FUNCTION_BLOCK FB_Visu
VAR_INPUT
	(***** Sensors to detect boxes *****)
	bBarrierSensor				AT %I*: BOOL;	// True if barrier sensor detects a box
	bMetalSensor				AT %I*: BOOL;	// True if metal sensor detects a metal box
	bPlasticSensor				AT %I*: BOOL;	// True if plastic sensor detects a box
	
	bError						: BOOL;			// True if modules have errors
(***** Axis variables *****)
	lrAxisVelo					: LREAL;
	
(***** State of machine elements *****)
	bComprAirEnabled			: BOOL;			// True if compressed air is enabled
	bPowerEnabled				: BOOL;			// True if power supply is enabled
	bMainAxisMoves				: BOOL;			// True if main axis is moving
	bMetalAxisMoves				: BOOL;			// True if metal axis is moving
	bPlasticAxisMoves			: BOOL;			// True if plastic axis is moving
	bClampToWork				: BOOL;			// True if clamp cylinder moves to work position
	bBarrierToWork				: BOOL;			// True if barrier cylinder moves to work position
	bMetalToWork				: BOOL;			// True if metal cylinder moves to work position
	bPlasticToWork				: BOOL;			// True if plastic cylinder moves to work position
(***** Error *****)
	bClampError					: BOOL;			// True if clamp cylinder has an error
	sClampErrMsg				: STRING;		// Error message of clamp cylinder
	bMetalCylError				: BOOL;			// True if metal cylinder has an error
	sMetalErrMsg				: STRING;		// Error message of metal cylinder
	bPlasticCylError			: BOOL;			// True if plastic cylinder has an error
	sPlasticErrMsg				: STRING;		// Error message of plastic cylinder
	nMainAxisErrorId			: DWORD;		// Error id of main axis
	nMetalAxisErrorId			: DWORD;		// Error id of metal axis
	nPlasticAxisErrorId			: DWORD;		// Error id of plastic axis
	
(***** PS_PackML_StateMachine *****)
	bStarted					: BOOL;			// True if state machine is in state EXECUTE
	bStopped					: BOOL;			// True if state machine is in state STOPPED
	bReset						: BOOL;			// True if state machine is in state RESETTING
	bAborted					: BOOL;			// True if state machine is in state ABORTED
	bIdle						: BOOL;			// True if state machine is in state IDLE
	bAuto						: BOOL;			// True if state machine is in mode AUTOMATIC
	bSemi						: BOOL;			// True if state machine is in mode SEMIAUTOMATIC
	bManual						: BOOL;			// True if state machine is in mode MANUAL
	bMaintenance				: BOOL;			// True if state machine is in mode MAINTENANCE
	bStartButtonOff				: BOOL;			// To turn off start button

(***** Buttons of visualisation - inputs *****)
		(* State buttons *)
	bButtonPowerIn				: BOOL;			// Input signal of power button
	bButtonComprAirIn			: BOOL;			// Input signal of compressed air button
	bButtonStartIn				: BOOL;			// Input signal of start button
	bButtonStopIn				: BOOL;			// Input signal of stop button
	bButtonResetIn				: BOOL;			// Input signal of reset button
	bButtonAbortIn				: BOOL;			// Input signal of abort button
		(* Mode buttons *)
	bButtonAutoIn				: BOOL;			// Input signal of automatic button
	bButtonSemiIn				: BOOL;			// Input signal of semi-automatic button
	bButtonManuIn				: BOOL;			// Input signal of manual button
	bButtonMaintenanceIn		: BOOL;			// Input signal of maintenance button
		(* Axis buttons *)
	bButtonMainFwIn				: BOOL;			// Input signal of button to move main axis forwards
	bButtonMainBwIn				: BOOL;			// Input signal of button to move main axis backwards
	bButtonMetalFwIn			: BOOL;			// Input signal of button to move metal axis forwards
	bButtonMetalBwIn			: BOOL;			// Input signal of button to move metal axis backwards
	bButtonPlasticFwIn			: BOOL;			// Input signal of button to move plastic axis forwards
	bButtonPlasticBwIn			: BOOL;			// Input signal of button to move plastic axis backwards
		(* Cylinder buttons *)
	bButtonClampToWorkIn		: BOOL;			// Input signal of button to move clamp cylinder
	bButtonBarrierToWorkIn		: BOOL;			// Input signal of button to move barrier cylinder
	bButtonMetalToWorkIn		: BOOL;			// Input signal of button to move metal cylinder
	bButtonPlasticToWorkIn		: BOOL;			// Input signal of button to move plastic cylinder
END_VAR
VAR_OUTPUT
	lrYClamp					AT %Q*: LREAL;					// Y-Coordinate of clamp cylinder
	lrYBarrier					AT %Q*: LREAL;					// Y-Coordinate of barrier cylinder
	lrYMetal					AT %Q*: LREAL;					// Y-Coordinate of metal cylinder
	lrYPlastic					AT %Q*: LREAL;					// Y-Coordinate of plastic cylinder
	aBoxX						AT %Q*: ARRAY[1..4] OF LREAL;	// X-Coordinates of boxes
	aBoxY						AT %Q*: ARRAY[1..4] OF LREAL;	// Y-Coordinates of boxes
	
(***** Buttons of visualisation - outputs *****)
		(* State buttons *)
	bButtonPowerOut				: BOOL;			// To turn on and off the machine
	bButtonComprAirOut			: BOOL;			// To enable compressed air
	bButtonStartOut				: BOOL;			// To change state into state START
	bButtonStopOut				: BOOL;			// To change state into state STOP
	bButtonResetOut				: BOOL;			// To change state into state RESET
	
		(* Mode buttons *)
	bButtonAutoOut				: BOOL;			// To change mode into mode AUTOMATIC		
	bButtonSemiOut				: BOOL;			// To change mode into mode SEMI-AUTOMATIC	
	bButtonManuOut				: BOOL;			// To change mode into mode MANAUL	
	bButtonMaintenanceOut		: BOOL;			// To change mode into mode MAINTENANCE	
	
		(* Axis buttons *)
	bButtonMainFwOut			: BOOL;			// To move main axis forwards
	bButtonMainBwOut			: BOOL;			// To move main axis backwards
	bButtonMetalFwOut			: BOOL;			// To move metal axis forwards
	bButtonMetalBwOut			: BOOL;			// To move metal axis backwards
	bButtonPlasticFwOut			: BOOL;			// To move plastic axis forwards
	bButtonPlasticBwOut			: BOOL;			// To move plastic axis backwards
	
		(* Cylinder buttons *)
	bButtonClampToWorkOut		: BOOL;			// To move manually clamp cylinder to work position
	bButtonBarrierToWorkOut		: BOOL;			// To move manually barrier cylinder to work position
	bButtonMetalToWorkOut		: BOOL;			// To move manually metal cylinder to work position
	bButtonPlasticToWorkOut		: BOOL;			// To move manually plastic cylinder to work position
END_VAR
VAR
	nBoxesLast					: INT;						// Box on last position of main belt
	aBoxMetalMove				: ARRAY[1..4] OF BOOL;		// bBoxMetalMove[1] is true, if box 1 is moved by metal cylinder
	aBoxMetalFree				: ARRAY[1..4] OF BOOL;		// bBoxMetalFree[1] is true, if any box blockades the metal belt
	aBoxPlasticMove				: ARRAY[1..4] OF BOOL;		// bBoxPlasticMove[1] is true, if box 1 is moved by plastic cylinder
	aBoxPlasticFree				: ARRAY[1..4] OF BOOL;		// bBoxMetalFree[1] is true, if any box blockades the plastic belt
	aBoxMainBelt				: ARRAY[1..4] OF BOOL;		// bBoxMainBelt[1] is true, if box 1 is on main belt and has no
	aBoxMetalBelt				: ARRAY[1..4] OF BOOL;				// obstacles, so box 1 is moved by main axis
	aBoxPlasticBelt				: ARRAY[1..4] OF BOOL;
	lrMainVelo					: LREAL;					// Velocity of boxes on main belt
	lrMetalVelo					: LREAL;					// Velocity of boxes on metal belt
	lrPlasticVelo				: LREAL;					// Velocity of boxes on plastic belt
	bAccident					: BOOL;						// True if machine caused an accident
	nState						: INT;
	
	nMessages					: INT;						// Number of messages
	sMessageClamp				: STRING;					// Message of clamp cylinder
	sMessageMetalCyl			: STRING;					// Message of metal cylinder
	sMessagePlasticCyl			: STRING;					// Message of plastic cylinder
	sMessageMainAxis			: STRING;					// Message of main axis
	sMessageMetalAxis			: STRING;					// Message of metal axis
	sMessagePlasticAxis			: STRING;					// Message of plastic axis
	nAngleMain					: INT;						// Angle of main axis element
	nAngleMetal					: INT;						// Angle of metal axis element
	nAnglePlastic				: INT;						// Angle of plastic axis element
	fbTimerMainAxis				: TON;						// Timer for movement of main axis element
	fbTimerMetalAxis			: TON;						// Timer for movement of metal axis element
	fbTimerPlasticAxis			: TON;						// Timer for movement of plastic axis element

(* ========================== COLOR VARIABLES =============================== *)

	nYellow						: DWORD;
	nGreen						: DWORD;
	nPink						: DWORD;
	nButtonColorStart			: DWORD;					// Color of start button
	bButtonColorStart			: BOOL;						// To change color of start button
	nButtonColorStop			: DWORD;					// Color of stop button
	bButtonColorStop			: BOOL;						// To change color of stop button
	nButtonColorReset			: DWORD;					// Color of reset button
	bButtonColorReset			: BOOL;						// To change color of reset button
	nButtonColorAuto			: DWORD;					// Color of automatic button
	bButtonColorAuto			: BOOL;						// To change color of automatic button
	nButtonColorSemi			: DWORD;					// Color of semi-automatic button
	bButtonColorSemi			: BOOL;						// To change color of semi-automatic button
	nButtonColorManu			: DWORD;					// Color of manual button
	bButtonColorManu			: BOOL;						// To change color of manual button
	nButtonColorMaint			: DWORD;					// Color of maintenance button
	bButtonColorMaint			: BOOL;						// To change color of maintenance button
	nButtonColorClamp			: DWORD;					// Color of button to move clamp cylinder
	bButtonColorClamp			: BOOL;						// To change color of clamp button
	nButtonColorBarrier			: DWORD;					// Color of button to move barrier cylinder
	bButtonColorBarrier			: BOOL;						// To change color of barrier button
	nButtonColorMetalCyl		: DWORD;					// Color of button to move metal cylinder
	bButtonColorMetalCyl		: BOOL;						// To change color of metal cylinder button
	nButtonColorPlasticCyl		: DWORD;					// Color of button to move plastic cylinder
	bButtonColorPlasticCyl		: BOOL;						// To change color of plastic cylinder button
	nButtonColorMainFw			: DWORD;					// Color of button to move main axis forwards
	bButtonColorMainFw			: BOOL;						// To change color of button to move main axis fw.
	nButtonColorMainBw			: DWORD;					// Color of button to move main axis backwards
	bButtonColorMainBw			: BOOL;						// To change color of button to move main axis bw.
	nButtonColorMetalFw			: DWORD;					// Color of button to move metal axis forwards
	bButtonColorMetalFw			: BOOL;						// To change color of button to move metal axis fw.
	nButtonColorMetalBw			: DWORD;					// Color of button to move metal axis backwards
	bButtonColorMetalBw			: BOOL;						// To change color of button to move metal axis bw.
	nButtonColorPlasticFw		: DWORD;					// Color of button to move plastic axis forwards
	bButtonColorPlasticFw		: BOOL;						// To change color of button to move plastic axis fw.
	nButtonColorPlasticBw		: DWORD;					// Color of button to move plastic axis backwards
	bButtonColorPlasticBw		: BOOL;						// To change color of button to move plastic axis bw.
	nButtonColorComprAir		: DWORD;					// Color of button to enable/disable compressed air
	bButtonColorComprAir		: BOOL;						// To change color of button to control compressed air
END_VAR

// =========================================================
	// Resetting visu
	
IF bReset THEN
	M_Reset();
END_IF

// =========================================================
	// Because of the visualisation size
	// the boxes velocity is a fraction of the axis velocity
	
IF bAuto OR bSemi OR bButtonMainFwIn THEN
	lrMainVelo := lrAxisVelo / 250;
ELSIF bButtonMainBwIn THEN
	lrMainVelo := - lrAxisVelo / 250;
END_IF

IF bAuto OR bSemi OR bButtonMetalFwIn THEN
	lrMetalVelo := - lrAxisVelo / 250;
ELSIF bButtonMetalBwIn THEN
	lrMetalVelo := lrAxisVelo / 250;
END_IF

IF bAuto OR bSemi OR bButtonPlasticFwIn THEN
	lrPlasticVelo := - lrAxisVelo / 250;
ELSIF bButtonPlasticBwIn THEN
	lrPlasticVelo := lrAxisVelo / 250;
END_IF

// =========================================================
	// In case of accident the power button is turned off
	
IF bAccident THEN
	IF bButtonPowerOut THEN
		bButtonPowerOut := FALSE;
	END_IF
	
	IF bStopped THEN
		bAccident := FALSE;
	END_IF
END_IF

// =========================================================
	// Rotation of axis elements
M_AxisRotation();

	// Buttons, order of boxes, error messages
M_ButtonSignals();
M_ButtonColors();
M_LastBox();
M_ErrorMessages();

	// Motion of cylinders
M_Barrier_Clamp_Cyl();
M_Metal_Plastic_Cyl();

	// Motion of boxes
M_AxisMoveBoxes();
M_CylinderMoveBoxes();

// =========================================================

METHOD PRIVATE M_ButtonSignals
VAR_INPUT
END_VAR
// =========================================================
	// When machine is in requested state, buttons are turned off again

IF bStartButtonOff THEN
	bButtonStartOut := FALSE;
END_IF

IF bStopped THEN
	bButtonStopOut := FALSE;
END_IF

IF bReset THEN
	bButtonResetOut := FALSE;
END_IF

IF bManual THEN
	bButtonManuOut := FALSE;
END_IF

IF bAuto THEN
	bButtonAutoOut := FALSE;
END_IF

IF bSemi THEN
	bButtonSemiOut := FALSE;
END_IF

IF bMaintenance THEN
	bButtonMaintenanceOut := FALSE;
END_IF

// =========================================================
END_METHOD

METHOD PRIVATE M_ButtonColors
VAR_INPUT
END_VAR
// =========================================================
		// Colors
		
nYellow := 16#00FFFF80;
nGreen 	:= 16#0080FF00;
nPink 	:= 16#00FF8080;

// =========================================================
		// Start button
		
IF (bAccident OR (bPowerEnabled AND (NOT bStarted OR (bSemi AND bStarted))
	AND NOT bButtonStopIn AND NOT bButtonAbortIn AND NOT bButtonResetIn
	AND (bAuto OR bSemi OR bManual OR bMaintenance))) AND NOT (bError AND bIdle) THEN
	
		IF bButtonStartOut THEN
			nButtonColorStart := nGreen;
		ELSE
			nButtonColorStart := nYellow;
		END_IF
		
		bButtonColorStart := TRUE;
ELSE
	bButtonColorStart := FALSE;
END_IF

// =========================================================
		// Stop button
		
IF (bStarted OR bIdle) AND (bAuto OR bSemi OR bManual OR bMaintenance) THEN
	IF bButtonStopOut THEN
		nButtonColorStop := nGreen;
	ELSE
		nButtonColorStop := nYellow;
	END_IF
	
	bButtonColorStop := TRUE;
ELSE
	bButtonColorStop := FALSE;
END_IF

// =========================================================
		// Reset button
		
IF bStopped AND bPowerEnabled THEN
	IF bButtonResetOut THEN
		nButtonColorReset := nGreen;
	ELSE
		nButtonColorReset := nYellow;		
	END_IF
	
	bButtonColorReset := TRUE;
ELSE
	bButtonColorReset := FALSE;
END_IF

// =========================================================
		// Mode buttons

IF bPowerEnabled THEN
	IF NOT bAuto THEN
		IF bIdle THEN
			nButtonColorAuto 	:= nYellow;
			bButtonColorAuto 	:= TRUE;
		ELSE
			bButtonColorAuto 	:= FALSE;
		END_IF
	ELSE
		nButtonColorAuto 		:= nGreen;
		bButtonColorAuto 		:= TRUE;
	END_IF
	
	IF NOT bSemi THEN
		IF bIdle THEN
			nButtonColorSemi 	:= nYellow;
			bButtonColorSemi 	:= TRUE;
		ELSE
			bButtonColorSemi 	:= FALSE;
		END_IF
	ELSE
		nButtonColorSemi 		:= nGreen;
		bButtonColorSemi 		:= TRUE;
	END_IF
	
	IF NOT bManual THEN
		IF bIdle THEN
			nButtonColorManu 	:= nYellow;
			bButtonColorManu 	:= TRUE;
		ELSE
			bButtonColorManu 	:= FALSE;
		END_IF
	ELSE
		nButtonColorManu 		:= nGreen;
		bButtonColorManu 		:= TRUE;
	END_IF
	
	IF NOT bMaintenance THEN
		IF bIdle THEN
			nButtonColorMaint 	:= nYellow;
			bButtonColorMaint 	:= TRUE;
		ELSE
			bButtonColorMaint 	:= FALSE;
		END_IF
	ELSE
		nButtonColorMaint 		:= nGreen;
		bButtonColorMaint 		:= TRUE;
	END_IF
END_IF

// =========================================================
		// Buttons to move cylinders and axes
		
IF (bManual OR bMaintenance) AND bStarted THEN
// Cylinders
	IF bButtonClampToWorkOut THEN
		nButtonColorClamp 	:= nPink;
	ELSE
		nButtonColorClamp 	:= nYellow;
	END_IF
	
	IF bButtonBarrierToWorkOut THEN
		nButtonColorBarrier := nPink;
	ELSE
		nButtonColorBarrier := nYellow;
	END_IF
	
	IF bButtonMetalToWorkOut THEN
		nButtonColorMetalCyl := nPink;
	ELSE
		nButtonColorMetalCyl := nYellow;
	END_IF
	
	IF bButtonPlasticToWorkOut THEN
		nButtonColorPlasticCyl := nPink;
	ELSE
		nButtonColorPlasticCyl := nYellow;
	END_IF
	
	bButtonColorClamp 		:= TRUE;
	bButtonColorBarrier 	:= TRUE;
	bButtonColorMetalCyl 	:= TRUE;
	bButtonColorPlasticCyl 	:= TRUE;
	
// Axes
	IF bButtonMainBwOut THEN
		nButtonColorMainBw := nPink;
	ELSE
		nButtonColorMainBw := nYellow;
	END_IF
	
	IF bButtonMainFwOut THEN
		nButtonColorMainFw := nPink;
	ELSE
		nButtonColorMainFw := nYellow;
	END_IF
	
	IF bButtonMetalBwOut THEN
		nButtonColorMetalBw := nPink;
	ELSE
		nButtonColorMetalBw := nYellow;
	END_IF
	
	IF bButtonMetalFwOut THEN
		nButtonColorMetalFw := nPink;
	ELSE
		nButtonColorMetalFw := nYellow;
	END_IF
	
	IF bButtonPlasticBwOut THEN
		nButtonColorPlasticBw := nPink;
	ELSE
		nButtonColorPlasticBw := nYellow;
	END_IF
	
	IF bButtonPlasticFwOut THEN
		nButtonColorPlasticFw := nPink;
	ELSE
		nButtonColorPlasticFw := nYellow;
	END_IF
	
	bButtonColorMainBw 		:= NOT bButtonMainFwOut;
	bButtonColorMainFw 		:= NOT bButtonMainBwOut;
	bButtonColorMetalBw 	:= NOT bButtonMetalFwOut;
	bButtonColorMetalFw 	:= NOT bButtonMetalBwOut;
	bButtonColorPlasticBw 	:= NOT bButtonPlasticFwOut;
	bButtonColorPlasticFw 	:= NOT bButtonPlasticBwOut;
ELSE
	bButtonColorClamp 		:= FALSE;
	bButtonColorBarrier 	:= FALSE;
	bButtonColorMetalCyl 	:= FALSE;
	bButtonColorPlasticCyl 	:= FALSE;
	bButtonColorMainBw 		:= FALSE;
	bButtonColorMainFw 		:= FALSE;
	bButtonColorMetalBw 	:= FALSE;
	bButtonColorMetalFw 	:= FALSE;
	bButtonColorPlasticBw 	:= FALSE;
	bButtonColorPlasticFw 	:= FALSE;
END_IF
		
// =========================================================
		// Button to control compressed air
		
IF bMaintenance AND bStarted THEN
	IF bButtonComprAirIn THEN
		nButtonColorComprAir := nGreen;
	ELSE
		nButtonColorComprAir := nYellow;
	END_IF
	
	bButtonColorComprAir := TRUE;
ELSE
	bButtonColorComprAir := FALSE;
END_IF

// =========================================================
END_METHOD

METHOD PRIVATE M_CylinderMoveBoxes
VAR_INPUT
END_VAR
// =========================================================
	// Metal cylinder - checking the positions of boxes
	
aBoxMetalFree[1] := NOT (aBoxX[2] > 300 AND aBoxX[2] <= 331 AND aBoxY[1] - aBoxY[2] <= 61)
					AND NOT (aBoxX[3] > 360 AND aBoxX[3] <= 391 AND aBoxY[1] - aBoxY[3] <= 61)
					AND NOT (aBoxX[4] > 420 AND aBoxX[4] <= 451 AND aBoxY[1] - aBoxY[4] <= 61);

aBoxMetalFree[2] := NOT (aBoxX[1] > 240 AND aBoxX[1] <= 271 AND aBoxY[2] - aBoxY[1] <= 61)
					AND NOT (aBoxX[3] > 360 AND aBoxX[3] <= 391 AND aBoxY[2] - aBoxY[3] <= 61)
					AND NOT (aBoxX[4] > 420 AND aBoxX[4] <= 451 AND aBoxY[2] - aBoxY[4] <= 61);
					
aBoxMetalFree[3] := NOT (aBoxX[1] > 240 AND aBoxX[1] <= 271 AND aBoxY[3] - aBoxY[1] <= 61)
					AND NOT (aBoxX[2] > 300 AND aBoxX[2] <= 331 AND aBoxY[3] - aBoxY[2] <= 61)
					AND NOT (aBoxX[4] > 420 AND aBoxX[4] <= 451 AND aBoxY[3] - aBoxY[4] <= 61);
					
aBoxMetalFree[4] := NOT (aBoxX[1] > 240 AND aBoxX[1] <= 271 AND aBoxY[4] - aBoxY[1] <= 61)
					AND NOT (aBoxX[2] > 300 AND aBoxX[2] <= 331 AND aBoxY[4] - aBoxY[2] <= 61)
					AND NOT (aBoxX[3] > 360 AND aBoxX[3] <= 391 AND aBoxY[4] - aBoxY[3] <= 61);

// =========================================================
	// Metal cylinder - boxes motion
	
FOR nState := 1 TO 4 BY 1 DO
	IF bMetalToWork AND aBoxMetalMove[nState] AND aBoxMetalFree[nState] THEN
		IF (lrYMetal - 1) >= -72 THEN
			lrYMetal := lrYMetal - 1;
			IF lrYMetal - aBoxY[nState] <= -9 THEN
				aBoxY[nState] := aBoxY[nState] - 1;
			END_IF
			
		ELSIF lrYMetal = -72 AND (lrYMetal - aBoxY[nState]) <= -9 THEN
			aBoxY[nState] := aBoxY[nState] - 2;
			
		ELSE
			aBoxMetalMove[nState] := FALSE;
		END_IF
	END_IF	
END_FOR

// =========================================================
// =========================================================
	// Plastic cylinder - checking the positions of boxes

aBoxPlasticFree[1] := NOT (aBoxX[2] > 550 AND aBoxX[2] <= 581 AND aBoxY[1] - aBoxY[2] <= 61)
					AND NOT (aBoxX[3] > 610 AND aBoxX[3] <= 641 AND aBoxY[1] - aBoxY[3] <= 61)
					AND NOT (aBoxX[4] > 670 AND aBoxX[4] <= 701 AND aBoxY[1] - aBoxY[4] <= 61);

aBoxPlasticFree[2] := NOT (aBoxX[1] > 490 AND aBoxX[1] <= 521 AND aBoxY[2] - aBoxY[1] <= 61)
					AND NOT (aBoxX[3] > 610 AND aBoxX[3] <= 641 AND aBoxY[2] - aBoxY[3] <= 61)
					AND NOT (aBoxX[4] > 670 AND aBoxX[4] <= 701 AND aBoxY[2] - aBoxY[4] <= 61);
					
aBoxPlasticFree[3] := NOT (aBoxX[1] > 490 AND aBoxX[1] <= 521 AND aBoxY[3] - aBoxY[1] <= 61)
					AND NOT (aBoxX[2] > 550 AND aBoxX[2] <= 581 AND aBoxY[3] - aBoxY[2] <= 61)
					AND NOT (aBoxX[4] > 670 AND aBoxX[4] <= 701 AND aBoxY[3] - aBoxY[4] <= 61);
					
aBoxPlasticFree[4] := NOT (aBoxX[1] > 490 AND aBoxX[1] <= 521 AND aBoxY[4] - aBoxY[1] <= 61)
					AND NOT (aBoxX[2] > 550 AND aBoxX[2] <= 581 AND aBoxY[4] - aBoxY[2] <= 61)
					AND NOT (aBoxX[3] > 610 AND aBoxX[3] <= 641 AND aBoxY[4] - aBoxY[3] <= 61);
					
// =========================================================
	// Plastic cylinder - boxes motion

FOR nState := 1 TO 4 BY 1 DO
	IF bPlasticToWork AND aBoxPlasticMove[nState] AND aBoxPlasticFree[nState] THEN
		IF (lrYPlastic - 1) >= -72 THEN
			lrYPlastic := lrYPlastic - 1;
			IF lrYPlastic - aBoxY[nState] <= -9 THEN
				aBoxY[nState] := aBoxY[nState] - 1;
			END_IF
			
		ELSIF lrYPlastic = -72 AND (lrYPlastic - aBoxY[nState]) <= -9 THEN
			aBoxY[nState] := aBoxY[nState] - 2;
			
		ELSE
			aBoxPlasticMove[nState] := FALSE;
		END_IF
	END_IF	
END_FOR

// =========================================================
END_METHOD

METHOD PRIVATE M_LastBox
VAR_INPUT
END_VAR
// =========================================================
	// Checking the last position on main belt

IF aBoxX[1] >= -180.05 AND aBoxX[1] < -120.05 AND aBoxY[1] = 0 THEN
	nBoxesLast := 1;
	
ELSIF aBoxX[2] >= -120.05 AND aBoxX[2] < -60.1 AND aBoxY[2] = 0 THEN
	nBoxesLast := 2;	
	
ELSIF aBoxX[3] >= -60.05 AND aBoxX[3] < -0.05 AND aBoxY[3] = 0 THEN
	nBoxesLast := 3;	
	
ELSIF aBoxX[4] >= -0.05 AND aBoxX[4] < 59.95 AND aBoxY[4] = 0 THEN
	nBoxesLast := 4;	
	
ELSE
	nBoxesLast := 0;
END_IF		

// =========================================================
END_METHOD

METHOD PRIVATE M_ErrorMessages
VAR_INPUT
END_VAR
// =========================================================
	// Error messages
	
nMessages := 0;
	
IF nMainAxisErrorId = 0 THEN
	sMessageMainAxis 	:= '';
ELSE
	nMessages 			:= nMessages + 1;
	sMessageMainAxis 	:= CONCAT('Error ID of main axis: ', DWORD_TO_STRING(nMainAxisErrorId));
END_IF
// =========================================================
IF nMetalAxisErrorId = 0 THEN
	sMessageMetalAxis 	:= '';
ELSE
	nMessages 			:= nMessages + 1;
	sMessageMetalAxis 	:= CONCAT('Error ID of metal axis: ', DWORD_TO_STRING(nMetalAxisErrorId));
END_IF
// =========================================================
IF nPlasticAxisErrorId = 0 THEN
	sMessagePlasticAxis	:= '';
ELSE
	nMessages 			:= nMessages + 1;
	sMessagePlasticAxis	:= CONCAT('Error ID of plastic axis: ', DWORD_TO_STRING(nPlasticAxisErrorId));
END_IF
// =========================================================
IF bClampError THEN
	nMessages 			:= nMessages + 1;
	sMessageClamp 		:= CONCAT('Error of clamp cylinder: ', sClampErrMsg);
ELSE
	sMessageClamp 		:= '';
END_IF
// =========================================================
IF bMetalCylError THEN
	nMessages 			:= nMessages + 1;
	sMessageMetalCyl 	:= CONCAT('Error of metal cylinder: ', sMetalErrMsg);
ELSE
	sMessageMetalCyl 	:= '';
END_IF
// =========================================================
IF bPlasticCylError THEN
	nMessages 			:= nMessages + 1;
	sMessagePlasticCyl 	:= CONCAT('Error of plastic cylinder: ', sPlasticErrMsg);
ELSE
	sMessagePlasticCyl 	:= '';
END_IF
// =========================================================
END_METHOD

METHOD PRIVATE M_Metal_Plastic_Cyl
VAR_INPUT
END_VAR
// =========================================================
	// Moving metal cylinder
	
IF bMetalToWork THEN
	IF NOT (aBoxMetalMove[1] OR aBoxMetalMove[2] OR aBoxMetalMove[3] OR aBoxMetalMove[4]) THEN
		IF (lrYMetal - 1) >= -73 THEN
			lrYMetal := lrYMetal - 1;
		END_IF
		
	ELSE
		FOR nState := 1 TO 4 BY 1 DO
			IF aBoxMetalMove[nState] THEN
				IF (lrYMetal - 1) >= (aBoxY[nState] - 9.1) AND (lrYMetal - 1) >= -73 THEN
					lrYMetal := lrYMetal - 1;
				END_IF
			END_IF
		END_FOR
	END_IF
	
ELSE
	IF (lrYMetal + 1) < 0.0 THEN
		lrYMetal := lrYMetal + 1;
	ELSE
		lrYMetal := 0.0;
	END_IF
END_IF

// =========================================================
	// Checking position of boxes related to the metal cylinder
	
IF lrYMetal < -8.9 AND lrYMetal > -9.1 AND bMetalToWork THEN
	FOR nState := 1 TO 4 BY 1 DO
			// box on main belt
		IF aBoxY[nState] >= -5 THEN
				// box in right position related to the metal cylinder
			IF aBoxX[nState] > (180 + 60*nState) AND aBoxX[nState] <= (211 + 60*nState) THEN
				aBoxMetalMove[nState] := TRUE;
			END_IF
				// box in wrong position related to the metal cylinder >> accident
			IF ((aBoxX[nState] > (131 + 60*nState) AND aBoxX[nState] <= (180 + 60*nState))
			OR (aBoxX[nState] > (211 + 60*nState) AND aBoxX[nState] < (261 + 60*nState)))
			AND NOT bStopped THEN
				bAccident := TRUE;
			END_IF
		END_IF
	END_FOR
END_IF

// =========================================================
// =========================================================
	// Moving plastic cylinder
	
IF bPlasticToWork THEN
	IF NOT (aBoxPlasticMove[1] OR aBoxPlasticMove[2] OR aBoxPlasticMove[3] OR aBoxPlasticMove[4]) THEN
		IF (lrYPlastic - 1) >= -73 THEN
			lrYPlastic := lrYPlastic - 1;
		END_IF
		
	ELSE
		FOR nState := 1 TO 4 BY 1 DO
			IF aBoxPlasticMove[nState] THEN
				IF (lrYPlastic - 1) >= (aBoxY[nState] - 9.1) AND (lrYPlastic - 1) >= -73 THEN
					lrYPlastic := lrYPlastic - 1;
				END_IF
			END_IF
		END_FOR
	END_IF
	
ELSE
	IF (lrYPlastic + 1) < 0 THEN
		lrYPlastic := lrYPlastic + 1;
	ELSE
		lrYPlastic := 0;
	END_IF
END_IF

// =========================================================
	// Checking position of boxes related to the plastic cylinder
	
IF (aBoxX[1] > 521 OR aBoxX[2] > 581 OR aBoxX[3] > 641 OR aBoxX[4] > 701)
AND NOT bStopped THEN
	bAccident := TRUE;
END_IF
	
IF lrYPlastic < -8.9 AND lrYPlastic > -9.1 AND bPlasticToWork THEN
	FOR nState := 1 TO 4 BY 1 DO
			// box on main belt
		IF aBoxY[nState] >= -5 THEN
				// box in right position related to the plastic cylinder
			IF aBoxX[nState] > (430 + 60*nState) AND aBoxX[nState] <= (461 + 60*nState) THEN
				aBoxPlasticMove[nState] := TRUE;
			END_IF
				// box in wrong position related to the plastic cylinder >> accident
			IF aBoxX[nState] > (381 + 60*nState) AND aBoxX[nState] <= (430 + 60*nState)
			AND NOT bStopped THEN
				bAccident := TRUE;
			END_IF	
		END_IF
	END_FOR
END_IF

// =========================================================
END_METHOD

METHOD PRIVATE M_Reset
VAR_INPUT
END_VAR
// =========================================================
	// Resetting visu
	
// Cylinder buttons
bButtonClampToWorkOut 		:= FALSE;
bButtonBarrierToWorkOut 	:= FALSE;
bButtonMetalToWorkOut 		:= FALSE;
bButtonPlasticToWorkOut 	:= FALSE;

// Axis buttons
bButtonMainBwOut 			:= FALSE;
bButtonMainFwOut 			:= FALSE;
bButtonMetalBwOut 			:= FALSE;
bButtonMetalFwOut 			:= FALSE;
bButtonPlasticBwOut			:= FALSE;
bButtonPlasticFwOut			:= FALSE;

// State and mode buttons
bButtonStartOut 			:= FALSE;
bButtonStopOut 				:= FALSE;
bButtonResetOut 			:= FALSE;
bButtonComprAirOut 			:= FALSE;
bButtonManuOut 				:= FALSE;
bButtonAutoOut 				:= FALSE;
bButtonSemiOut 				:= FALSE;
bButtonMaintenanceOut		:= FALSE;

// Position of boxes and cylinders	
FOR nState := 1 TO 4 BY 1 DO
	aBoxX[nState] 			:= 0;
	aBoxY[nState] 			:= 0;
	
	aBoxMetalMove[nState] 	:= FALSE;
	aBoxPlasticMove[nState]	:= FALSE;
	aBoxMainBelt[nState]	:= FALSE;
	aBoxMetalBelt[nState] 	:= FALSE;
	aBoxPlasticBelt[nState]	:= FALSE;
END_FOR

bAccident := FALSE;

// =========================================================
END_METHOD

METHOD PRIVATE M_AxisMoveBoxes
VAR_INPUT
END_VAR
// =========================================================
	// Checking traction standby on main belt
	
aBoxMainBelt[1] := aBoxY[1] >= -5	// box 1 on main belt
						// not previous to box 2											
					AND ((aBoxX[2] - aBoxX[1] - lrMainVelo) >= 119.99999 OR (aBoxX[2] - aBoxX[1] - lrMainVelo) <= 0.001 OR aBoxY[2] < -60)
						// not previous to box 3	
					AND ((aBoxX[3] - aBoxX[1] - lrMainVelo) >= 179.99999 OR (aBoxX[3] - aBoxX[1]- lrMainVelo) <= 60.001 OR aBoxY[3] < -60)
						// not previous to box 4
					AND ((aBoxX[4] - aBoxX[1] - lrMainVelo) >= 239.99999 OR (aBoxX[4] - aBoxX[1]- lrMainVelo) <= 120.001 OR aBoxY[4] < -60);
					
aBoxMainBelt[2] := aBoxY[2] >= -5
					AND ((aBoxX[1] - aBoxX[2] - lrMainVelo) >= -0.00001 OR (aBoxX[1] - aBoxX[2] - lrMainVelo) <= -119.999 OR aBoxY[1] < -60)
					AND ((aBoxX[3] - aBoxX[2] - lrMainVelo) >= 119.99999 OR (aBoxX[3] - aBoxX[2] - lrMainVelo) <= 0.001 OR aBoxY[3] < -60)
					AND ((aBoxX[4] - aBoxX[2] - lrMainVelo) >= 179.99999 OR (aBoxX[4] - aBoxX[2] - lrMainVelo) <= 60.001 OR aBoxY[4] < -60);

aBoxMainBelt[3] := aBoxY[3] >= -5
					AND ((aBoxX[1] - aBoxX[3] - lrMainVelo) >= -60.00001 OR (aBoxX[1] - aBoxX[3] - lrMainVelo) <= -179.999 OR aBoxY[1] < -60)
					AND ((aBoxX[2] - aBoxX[3] - lrMainVelo) >= -0.00001 OR (aBoxX[2] - aBoxX[3] - lrMainVelo) <= -119.999 OR aBoxY[2] < -60)
					AND ((aBoxX[4] - aBoxX[3] - lrMainVelo) >= 119.99999 OR (aBoxX[4] - aBoxX[3] - lrMainVelo) <= 0.001 OR aBoxY[4] < -60);
					
aBoxMainBelt[4] := aBoxY[4] >= -5
					AND ((aBoxX[1] - aBoxX[4] - lrMainVelo) >= -120.00001 OR (aBoxX[1] - aBoxX[4] - lrMainVelo) <= -239.999 OR aBoxY[1] < -60)
					AND ((aBoxX[2] - aBoxX[4] - lrMainVelo) >= -60.00001 OR (aBoxX[2] - aBoxX[4] - lrMainVelo) <= -179.999 OR aBoxY[2] < -60)
					AND ((aBoxX[3] - aBoxX[4] - lrMainVelo) >= -0.00001 OR (aBoxX[3] - aBoxX[4] - lrMainVelo) <= -119.999 OR aBoxY[3] < -60);
					
// =========================================================
	// Motion of boxes on main belt - forwards
					
IF bMainAxisMoves AND (bAuto OR bSemi OR bButtonMainFwIn) THEN
	FOR nState := 1 TO 4 BY 1 DO
		IF aBoxMainBelt[nState] THEN	
				// not previous to moving metal cylinder
			IF aBoxX[nState] >= (60*nState + 30) AND aBoxX[nState] < (260 + 60*nState) THEN
				IF lrYMetal <= -9 THEN
					IF aBoxX[nState] < (131.25 + 60*nState) AND aBoxX[nState] > (130.95 + 60*nState) THEN
						aBoxX[nState] := 131 + 60*nState;
					ELSIF aBoxX[nState] <= (130.95 + 60*nState) THEN
						aBoxX[nState] := aBoxX[nState] + lrMainVelo;
					END_IF
				ELSE
					aBoxX[nState] := aBoxX[nState] + lrMainVelo;
				END_IF
			END_IF
				// not previous to moving plastic cylinder
			IF aBoxX[nState] >= (260 + 60*nState) THEN
				IF lrYPlastic <= -9 THEN
					IF aBoxX[nState] < (381.25 + 60*nState) AND aBoxX[nState] > (380.95 + 60*nState) THEN
						aBoxX[nState] := 381 + 60*nState;
					ELSIF aBoxX[nState] <= (380.95 + 60*nState) THEN
						aBoxX[nState] := aBoxX[nState] + lrMainVelo;
					END_IF
				ELSE
					aBoxX[nState] := aBoxX[nState] + lrMainVelo;
				END_IF
			END_IF
				// barrier open and box 1 in the first place
			IF lrYBarrier >= 61 AND aBoxX[nState] >= 60*(nState - 1) AND aBoxX[nState] <  (60*nState + 30) THEN
				IF aBoxX[nState] + lrMainVelo < (60*nState + 30) THEN
					 aBoxX[nState] := aBoxX[nState] + lrMainVelo;
				ELSIF aBoxX[nState] < (60*nState + 30) THEN
					aBoxX[nState] := (60*nState + 30);
				END_IF
			END_IF	
				// not previous to clamp
			IF aBoxX[nState] + lrMainVelo < -60*(3 - nState) THEN
				aBoxX[nState] := aBoxX[nState] + lrMainVelo;
			ELSIF aBoxX[nState] < -60*(nState + 1) THEN
				aBoxX[nState] := -60*(nState + 1);
			END_IF
				// clamp open, not after clamp											
			IF lrYClamp >= 1 AND aBoxX[nState] >= -60*(nState + 1) THEN
				IF aBoxX[nState] + lrMainVelo < 60*(nState - 1) THEN
					aBoxX[nState] := aBoxX[nState] + lrMainVelo;
				ELSIF aBoxX[nState] < 60*(nState - 1) THEN
					aBoxX[nState] := 60*(nState - 1);
				END_IF
			END_IF
		END_IF
	END_FOR
END_IF

// =========================================================
	// Motion of boxes on main belt - backwards
	
IF bMainAxisMoves AND bButtonMainBwIn THEN 
	FOR nState := 1 TO 4 BY 1 DO
		IF aBoxMainBelt[nState] THEN
				// not previous to moving metal cylinder
			IF aBoxX[nState] >= (90 + 60*nState) AND aBoxX[nState] < (262 + 60*nState) THEN
				IF NOT (aBoxX[nState] < (261.25 + 60*nState) AND aBoxX[nState] > (260.95 + 60*nState) AND lrYMetal <= -9) THEN
					aBoxX[nState] := aBoxX[nState] + lrMainVelo;
				ELSE
					aBoxX[nState] := 261 + 60*nState;
				END_IF
			END_IF
				// not previous to moving plastic cylinder
			IF aBoxX[nState] >=  (262 + 60*nState) THEN
				aBoxX[nState] := aBoxX[nState] + lrMainVelo;
			END_IF
				// not previous to moving barrier cylinder
			IF aBoxX[nState] > 60*(nState - 1) AND aBoxX[nState] < (90 + 60*nState) THEN
				IF NOT (aBoxX[nState] < (30.25 + 60*nState) AND aBoxX[nState] > (29.95 + 60*nState) AND lrYBarrier < 61) THEN
					aBoxX[nState] := aBoxX[nState] + lrMainVelo;
				ELSE
					aBoxX[nState] := 60*nState + 30;
				END_IF
			END_IF
				// barrier open and box 1 after the first place
			IF lrYBarrier >= 61 AND aBoxX[nState] < 60*(nState + 1) AND aBoxX[nState] > 60*(nState - 1) THEN
				aBoxX[nState] := aBoxX[nState] + lrMainVelo;
			END_IF	
				// clamp open, not previous to clamp											
			IF lrYClamp >= 1 AND aBoxX[nState] <= 60*(nState-1) AND aBoxX[nState] > -60*(3-nState) THEN
				aBoxX[nState] := aBoxX[nState] + lrMainVelo;
			END_IF
				// not at the beginning of main belt
			IF aBoxX[nState] > -60*(4-nState) AND aBoxX[nState] <= -60*(3-nState) THEN
				aBoxX[nState] := aBoxX[nState] + lrMainVelo;
			END_IF
		END_IF
	END_FOR	
END_IF

// =========================================================
// =========================================================
	// Checking traction standby on metal belt
	
aBoxMetalBelt[1] := aBoxX[1] > 240 AND aBoxX[1] <= 271	// box 1 on metal belt
						// not previous to box 2											
					AND ((aBoxY[2] - aBoxY[1] - lrMetalVelo) >= 60 OR (aBoxY[2] - aBoxY[1] - lrMetalVelo) <= -60
							OR NOT (aBoxX[2] > 300 AND aBoxX[2] <= 331))
						// not previous to box 3	
					AND ((aBoxY[3] - aBoxY[1]- lrMetalVelo) >= 60 OR (aBoxY[3] - aBoxY[1]- lrMetalVelo) <= -60
							OR NOT (aBoxX[3] > 360 AND aBoxX[3] <= 391))
						// not previous to box 4
					AND ((aBoxY[4] - aBoxY[1]- lrMetalVelo) >= 60 OR (aBoxY[4] - aBoxY[1]- lrMetalVelo) <= -60
							OR NOT (aBoxX[4] > 420 AND aBoxX[4] <= 451));	
					
aBoxMetalBelt[2] := aBoxX[2] > 300 AND aBoxX[2] <= 331										
					AND ((aBoxY[1] - aBoxY[2] - lrMetalVelo) >= 60 OR (aBoxY[1] - aBoxY[2] - lrMetalVelo) <= -60
							OR NOT (aBoxX[1] > 240 AND aBoxX[1] <= 271))
					AND ((aBoxY[3] - aBoxY[2]- lrMetalVelo) >= 60 OR (aBoxY[3] - aBoxY[2]- lrMetalVelo) <= -60
							OR NOT (aBoxX[3] > 360 AND aBoxX[3] <= 391))
					AND ((aBoxY[4] - aBoxY[2]- lrMetalVelo) >= 60 OR (aBoxY[4] - aBoxY[2]- lrMetalVelo) <= -60
							OR NOT (aBoxX[4] > 420 AND aBoxX[4] <= 451));	
					
aBoxMetalBelt[3] := aBoxX[3] > 360 AND aBoxX[3] <= 391										
					AND ((aBoxY[1] - aBoxY[3] - lrMetalVelo) >= 60 OR (aBoxY[1] - aBoxY[3] - lrMetalVelo) <= -60
							OR NOT (aBoxX[1] > 240 AND aBoxX[1] <= 271))
					AND ((aBoxY[2] - aBoxY[3]- lrMetalVelo) >= 60 OR (aBoxY[2] - aBoxY[3]- lrMetalVelo) <= -60
							OR NOT (aBoxX[2] > 300 AND aBoxX[2] <= 331))
					AND ((aBoxY[4] - aBoxY[3]- lrMetalVelo) >= 60 OR (aBoxY[4] - aBoxY[3]- lrMetalVelo) <= -60
							OR NOT (aBoxX[4] > 420 AND aBoxX[4] <= 451));	
					
aBoxMetalBelt[4] := aBoxX[4] > 420 AND aBoxX[4] <= 451										
					AND ((aBoxY[1] - aBoxY[4] - lrMetalVelo) >= 60 OR (aBoxY[1] - aBoxY[4] - lrMetalVelo) <= -60
							OR NOT (aBoxX[1] > 240 AND aBoxX[1] <= 271))
					AND ((aBoxY[2] - aBoxY[4] - lrMetalVelo) >= 60 OR (aBoxY[2] - aBoxY[4] - lrMetalVelo) <= -60
							OR NOT (aBoxX[2] > 300 AND aBoxX[2] <= 331))
					AND ((aBoxY[3] - aBoxY[4]- lrMetalVelo) >= 60 OR (aBoxY[3] - aBoxY[4]- lrMetalVelo) <= -60
							OR NOT (aBoxX[3] > 360 AND aBoxX[3] <= 391));

// =========================================================
	// Motion of boxes on metal belt and back to the start position number 4
	
FOR nState := 1 TO 4 BY 1 DO	
	IF bMetalAxisMoves THEN
		IF 	aBoxMetalBelt[nState] THEN
		(* Check the state and direction of motion *)		
				IF bAuto OR bSemi OR (NOT bAuto AND bButtonMetalFwIn) THEN
				(* Move box to the end of metal belt and then back to position 4 *)	
					IF aBoxY[nState] <= -64.9 AND aBoxY[nState] > -140.0 THEN
						aBoxY[nState] := aBoxY[nState] + lrMetalVelo;
					END_IF
					
				ELSIF NOT bAuto AND bButtonMetalBwIn THEN
					IF aBoxY[nState] + lrMetalVelo <= -65.1 THEN
						aBoxY[nState] := aBoxY[nState] + lrMetalVelo;
					END_IF
				END_IF
		END_IF
	END_IF	
	
	IF aBoxY[nState] <= -140.0 AND nBoxesLast = 0 THEN
		aBoxY[nState] := 0;
		aBoxX[nState] := -240 + nState*60;
	END_IF
END_FOR
	
// =========================================================
// =========================================================
	// Checking traction standby on plastic belt
	
aBoxPlasticBelt[1] := aBoxX[1] > 470 AND aBoxX[1] <= 521	// box 1 on plastic belt
						// not previous to box 2											
					AND ((aBoxY[2] - aBoxY[1] - lrPlasticVelo) >= 60 OR (aBoxY[2] - aBoxY[1] - lrPlasticVelo) <= -60
							OR NOT (aBoxX[2] > 530 AND aBoxX[2] <= 581))
						// not previous to box 3	
					AND ((aBoxY[3] - aBoxY[1]- lrPlasticVelo) >= 60 OR (aBoxY[3] - aBoxY[1]- lrPlasticVelo) <= -60
							OR NOT (aBoxX[3] > 590 AND aBoxX[3] <= 641))
						// not previous to box 4
					AND ((aBoxY[4] - aBoxY[1]- lrPlasticVelo) >= 60 OR (aBoxY[4] - aBoxY[1]- lrPlasticVelo) <= -60
							OR NOT (aBoxX[4] > 650 AND aBoxX[4] <= 701));	
					
aBoxPlasticBelt[2] := aBoxX[2] > 530 AND aBoxX[2] <= 581										
					AND ((aBoxY[1] - aBoxY[2] - lrPlasticVelo) >= 60 OR (aBoxY[1] - aBoxY[2] - lrPlasticVelo) <= -60
							OR NOT (aBoxX[1] > 470 AND aBoxX[1] <= 521))
					AND ((aBoxY[3] - aBoxY[2]- lrPlasticVelo) >= 60 OR (aBoxY[3] - aBoxY[2]- lrPlasticVelo) <= -60
							OR NOT (aBoxX[3] > 590 AND aBoxX[3] <= 641))
					AND ((aBoxY[4] - aBoxY[2]- lrPlasticVelo) >= 60 OR (aBoxY[4] - aBoxY[2]- lrPlasticVelo) <= -60
							OR NOT (aBoxX[4] > 650 AND aBoxX[4] <= 701));	
					
aBoxPlasticBelt[3] := aBoxX[3] > 590 AND aBoxX[3] <= 641										
					AND ((aBoxY[1] - aBoxY[3] - lrPlasticVelo) >= 60 OR (aBoxY[1] - aBoxY[3] - lrPlasticVelo) <= -60
							OR NOT (aBoxX[1] > 470 AND aBoxX[1] <= 521))
					AND ((aBoxY[2] - aBoxY[3]- lrPlasticVelo) >= 60 OR (aBoxY[2] - aBoxY[3]- lrPlasticVelo) <= -60
							OR NOT (aBoxX[2] > 530 AND aBoxX[2] <= 581))
					AND ((aBoxY[4] - aBoxY[3]- lrPlasticVelo) >= 60 OR (aBoxY[4] - aBoxY[3]- lrPlasticVelo) <= -60
							OR NOT (aBoxX[4] > 650 AND aBoxX[4] <= 701));	
					
aBoxPlasticBelt[4] := aBoxX[4] > 650 AND aBoxX[4] <= 701										
					AND ((aBoxY[1] - aBoxY[4] - lrPlasticVelo) >= 60 OR (aBoxY[1] - aBoxY[4] - lrPlasticVelo) <= -60
							OR NOT (aBoxX[1] > 470 AND aBoxX[1] <= 521))
					AND ((aBoxY[2] - aBoxY[4] - lrPlasticVelo) >= 60 OR (aBoxY[2] - aBoxY[4] - lrPlasticVelo) <= -60
							OR NOT (aBoxX[2] > 530 AND aBoxX[2] <= 581))
					AND ((aBoxY[3] - aBoxY[4]- lrPlasticVelo) >= 60 OR (aBoxY[3] - aBoxY[4]- lrPlasticVelo) <= -60
							OR NOT (aBoxX[3] > 590 AND aBoxX[3] <= 641));

// =========================================================
	// Motion of boxes on metal belt and back to the start position number 4

FOR nState := 1 TO 4 BY 1 DO	
	IF bPlasticAxisMoves THEN
			IF 	aBoxPlasticBelt[nState] THEN	
				(* Check the state and direction of motion *)		
				IF bAuto OR bSemi OR (NOT bAuto AND bButtonPlasticFwIn) THEN
				(* Move box to the end of metal belt and then back to position 4 *)	
					IF aBoxY[nState] <= -64.9 AND aBoxY[nState] > -140.0 THEN
						aBoxY[nState] := aBoxY[nState] + lrPlasticVelo;
					END_IF
					
				ELSIF NOT bAuto AND bButtonPlasticBwIn THEN
					IF aBoxY[nState] + lrPlasticVelo <= -65.1 THEN
						aBoxY[nState] := aBoxY[nState] + lrPlasticVelo;
					END_IF
				END_IF
			END_IF
	END_IF
	
	IF aBoxY[nState] <= -140.0 AND nBoxesLast = 0 THEN
		aBoxY[nState] := 0;
		aBoxX[nState] := -240 + nState*60;
	END_IF
END_FOR

// =========================================================
END_METHOD

METHOD PRIVATE M_AxisRotation
VAR_INPUT
END_VAR
// =========================================================
	// Rotation of main axis
	
fbTimerMainAxis(IN := bMainAxisMoves,
			 	PT := T#0.04S );

IF fbTimerMainAxis.Q THEN
	fbTimerMainAxis( IN := FALSE );
	
	IF bAuto OR bSemi THEN
		nAngleMain := nAngleMain + 2;
		
	ELSIF bButtonMainFwIn THEN
		nAngleMain := nAngleMain + 1;
		
	ELSIF bButtonMainBwIn THEN
		nAngleMain := nAngleMain - 1;
	END_IF
END_IF

// =========================================================
	// Rotation of metal axis
	
fbTimerMetalAxis( 	IN := bMetalAxisMoves,
			 		PT := T#0.04S );

IF fbTimerMetalAxis.Q THEN
	fbTimerMetalAxis( IN := FALSE );
	
	IF bAuto OR bSemi THEN
		nAngleMetal := nAngleMetal + 2;
		
	ELSIF bButtonMetalFwIn THEN
		nAngleMetal := nAngleMetal + 1;
		
	ELSIF bButtonMetalBwIn THEN
		nAngleMetal := nAngleMetal - 1;
	END_IF
END_IF

// =========================================================
	// Rotation of plastic axis
	
fbTimerPlasticAxis( IN := bPlasticAxisMoves,
					PT := T#0.04S );

IF fbTimerPlasticAxis.Q THEN
	fbTimerPlasticAxis( IN := FALSE );
	
	IF bAuto OR bSemi THEN
		nAnglePlastic := nAnglePlastic + 2;
		
	ELSIF bButtonPlasticFwIn THEN
		nAnglePlastic := nAnglePlastic + 1;
		
	ELSIF bButtonPlasticBwIn THEN
		nAnglePlastic := nAnglePlastic - 1;
	END_IF
END_IF

// =========================================================
END_METHOD

METHOD PRIVATE M_Barrier_Clamp_Cyl
VAR_INPUT
END_VAR
// =========================================================
	// Moving clamp cylinder
	
IF bClampToWork THEN
	IF (lrYClamp + 0.1) < 3.0 THEN
		lrYClamp := lrYClamp + 0.1;
	ELSE
		lrYClamp := 3.0;
	END_IF
	
ELSE
	IF (lrYClamp - 0.1) > 0.0 THEN
		lrYClamp := lrYClamp - 0.1;
	ELSE
		lrYClamp := 0.0;
	END_IF
END_IF

// =========================================================
// =========================================================
	// Moving barrier cylinder
	
IF bBarrierToWork THEN
	IF (lrYBarrier + 1) < 63.0 THEN
		lrYBarrier := lrYBarrier + 1;
	ELSE
		lrYBarrier := 63.0;
	END_IF
	
ELSE
	IF (lrYBarrier - 1) > 0.0 THEN
		lrYBarrier := lrYBarrier - 1;
	ELSE
		lrYBarrier := 0.0;
	END_IF
END_IF

// =========================================================
	// Checking position of boxes related to the barrier cylinder
	
IF lrYBarrier <= 60 AND NOT bBarrierToWork THEN
	
	FOR nState := 1 TO 4 BY 1 DO
		IF aBoxX[nState] > (-59.89 + 60*nState) AND aBoxX[nState] < (60*nState + 30) AND aBoxY[nState] = 0
			AND NOT bStopped THEN
				bAccident := TRUE;
		END_IF
	END_FOR
	
END_IF

// =========================================================
END_METHOD

END_FUNCTION_BLOCK
